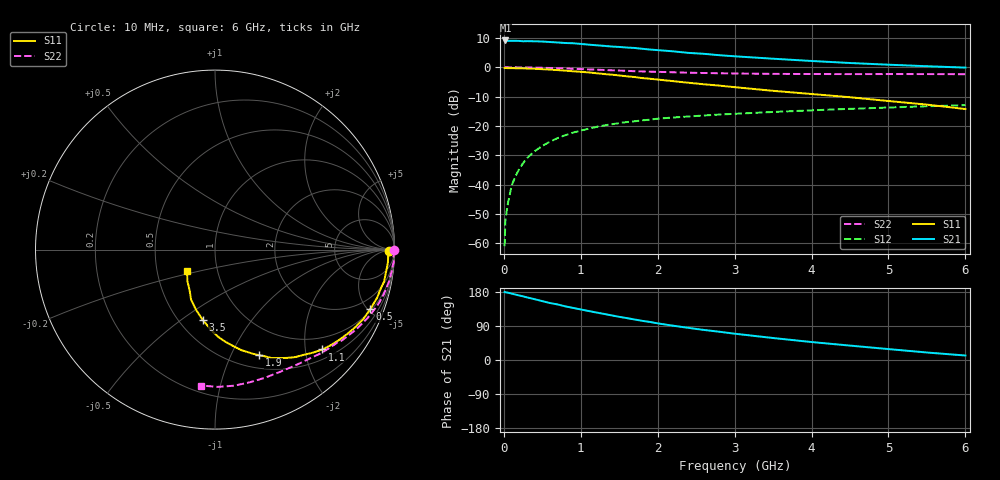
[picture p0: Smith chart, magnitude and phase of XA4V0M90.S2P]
! SIEMENS Discrete & RF Semiconductors
! BFY180
! Si NPN RF Bipolar Junction Transistor in MICRO-X
! VCE = 4 V  IC = 0.9 mA
! Common Emitter S-Parameters:  May  1997
# GHz  S  MA  R  50
!  f  S11  S21  S12  S22
! GHz  MAG  ANG  MAG  ANG  MAG  ANG  MAG  ANG
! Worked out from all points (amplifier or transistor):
!   36 points, 10 MHz to 6 GHz, reference 50 ohm
!   highest |S21| = 9.1 dB at 20 MHz (marker M1)
!   |S21| within 3 dB of that: start of sweep to 1.864 GHz
!   unconditionally stable (mu >= 1): 4.195 GHz to end of sweep
!   at 250 MHz: K = 0.07, MSG = 20.7 dB, |S12| = -32.7 dB
!   at 1.4 GHz: K = 0.47, MSG = 13.2 dB, |S12| = -19.4 dB
!   at 6 GHz: K = 1.05, MAG = 5.0 dB, |S12| = -12.9 dB
!   S11 on the Smith chart (normalised r, x): 10 MHz: 61, -10; 500 MHz: 1.10, -5.17; 1.1 GHz: 0.71, -2.36; 1.9 GHz: 0.65, -1.28; 3.5 GHz: 0.65, -0.60; 6 GHz: 0.71, -0.17
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0.01  0.9686 -0.3  2.81 179.6  0.0009 81.0  0.9985 -0.2
0.02  0.9702 -0.7  2.858 178.7  0.0025 87.4  0.9991 -0.5
0.05  0.9658 -2.1  2.818 177.7  0.0046 84.8  0.9977 -1.2
0.1  0.9659 -4.4  2.817 175.3  0.0095 87.0  0.9947 -2.6
0.15  0.9624 -6.5  2.816 172.8  0.0139 86.6  0.9987 -3.9
0.3  0.9507 -12.6  2.781 165.3  0.0283 81.1  0.9901 -7.7
0.5  0.9266 -21.0  2.74 155.4  0.0458 75.6  0.9789 -12.7
0.6  0.9131 -24.9  2.687 150.3  0.0541 72.7  0.9716 -15.1
0.8  0.8748 -32.4  2.586 141.5  0.0698 67.1  0.9527 -19.8
0.9  0.8542 -36.3  2.562 137.5  0.0772 63.8  0.9412 -22.1
1.1  0.8172 -42.9  2.427 129.4  0.0897 59.4  0.9192 -26.2
1.5  0.7253 -56.3  2.216 113.9  0.112 51.0  0.8779 -33.9
1.7  0.6812 -62.5  2.129 106.9  0.1203 47.5  0.8554 -37.3
1.9  0.6371 -67.4  2.002 100.4  0.1283 44.3  0.8405 -40.6
2.2  0.5798 -75.2  1.867 90.5  0.1394 40.2  0.8215 -45.2
2.6  0.5132 -84.1  1.693 79.3  0.1509 35.5  0.7981 -50.7
3  0.458 -91.6  1.537 69.4  0.1612 31.4  0.7831 -56.0
3.5  0.3969 -100.0  1.397 58.0  0.1733 27.3  0.7713 -62.2
4  0.35 -107.8  1.279 47.4  0.1848 23.0  0.7664 -68.7
4.5  0.3086 -115.6  1.181 38.0  0.1959 19.1  0.7643 -75.2
5.5  0.2311 -132.0  1.041 19.8  0.2168 11.3  0.765 -88.9
6  0.1944 -142.9  0.986 11.8  0.226 7.0  0.7614 -95.9
